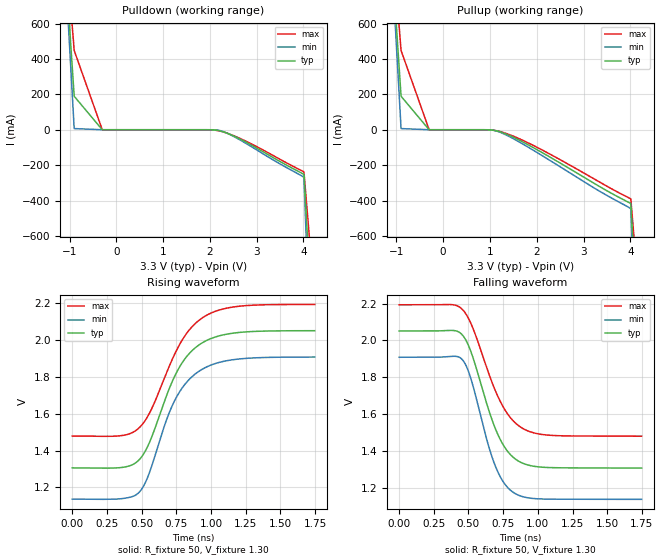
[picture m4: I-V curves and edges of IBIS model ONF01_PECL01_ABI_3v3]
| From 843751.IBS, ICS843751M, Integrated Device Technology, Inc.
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[Model] ONF01_PECL01_ABI_3v3
Model_type   Output_ECL
Polarity   Non-Inverting
|   typ   min   max
C_comp   2pF   1.5pF   2.5pF
Vmeas = 1.62V
Rref = 50
Cref = 0
Vref = 1.3V
|   typ   min   max
[Voltage range]   3.3V   3.135V   3.465V
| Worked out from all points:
|   rising waveform, R_fixture 50, V_fixture 1.30: 20-80 % time 253ps typ, 244ps min, 269ps max; typ from 1.31 V to 2.05 V
|   falling waveform, R_fixture 50, V_fixture 1.30: 20-80 % time 199ps typ, 176ps min, 223ps max; typ from 2.05 V to 1.31 V
[Pulldown]
|Voltage   I (typ)   I (min)   I (max)
-3.3V     9.786A     12.03A     8.45A
-1.5V     2.58A      2.839A     2.441A
-900mV    189.2mA    6.554mA    448mA
-300mV    38.6nA     139.1pA    1.11uA
1.978V    -80.11uA   -13.25uA   -238.1uA
2.126V    -1.925mA   -870.5uA   -2.993mA
2.274V    -10.73mA   -9.534mA   -11.63mA
2.471V    -31.01mA   -32.89mA   -29.75mA
2.817V    -76.79mA   -84.38mA   -70.9mA
4.01V     -252.1mA   -270.1mA   -237.9mA
4.528V    -2.68A     -3.925A    -1.887A
6.6V      -15.69A    -20.55A    -12.73A
[Pullup]
|Voltage   I (typ)   I (min)   I (max)
-3.3V     9.786A     12.03A     8.45A
-1.5V     2.58A      2.839A     2.441A
-900mV    189.2mA    6.554mA    448mA
-300mV    38.6nA     139.1pA    1.11uA
1.041V    -1.682mA   -1.459mA   -1.692mA
1.288V    -18.79mA   -22.48mA   -15.95mA
1.682V    -66.58mA   -77.82mA   -57.47mA
2.274V    -153.4mA   -172.3mA   -136.7mA
3.26V     -308.2mA   -334.6mA   -283.1mA
4.01V     -417.2mA   -447.3mA   -390.7mA
4.528V    -2.844A    -4.101A    -2.04A
6.6V      -15.79A    -20.6A     -12.84A
[Ramp]
|   typ   min   max
dV/dt_r   0.597/0.406n   0.618/0.395n   0.573/0.427n
dV/dt_f   0.598/0.304n   0.622/0.269n   0.572/0.341n
R_load =   50.0000
[Rising Waveform]
R_fixture = 50
V_fixture = 1.30   | VCC_typ - 2V
V_fixture_max = 1.465   | VCC_max - 2V
V_fixture_min = 1.135   | VCC_min - 2V
C_fixture = 0.0p
| Time   typ   min   max
0s        1.306V     1.136V     1.479V
348.6ps   1.308V     1.138V     1.481V
480ps     1.348V     1.172V     1.522V
546.5ps   1.427V     1.261V     1.589V
672.7ps   1.684V     1.553V     1.81V
741ps     1.808V     1.676V     1.929V
828.6ps   1.914V     1.775V     2.041V
933.7ps   1.984V     1.841V     2.119V
1.184ns   2.04V      1.896V     2.183V
1.748ns   2.051V     1.908V     2.194V
[Falling Waveform]
R_fixture = 50
V_fixture = 1.30   | VCC_typ - 2V
V_fixture_max = 1.465   | VCC_max - 2V
V_fixture_min = 1.135   | VCC_min - 2V
C_fixture = 0.0p
| Time   typ   min   max
0s        2.052V     1.909V     2.194V
380.1ps   2.055V     1.914V     2.195V
457.2ps   2.029V     1.894V     2.168V
516.8ps   1.94V      1.794V     2.093V
634.1ps   1.65V      1.454V     1.846V
691.9ps   1.524V     1.32V      1.73V
756.8ps   1.424V     1.224V     1.63V
833.8ps   1.358V     1.169V     1.554V
1.053ns   1.31V      1.138V     1.487V
1.748ns   1.306V     1.136V     1.479V
